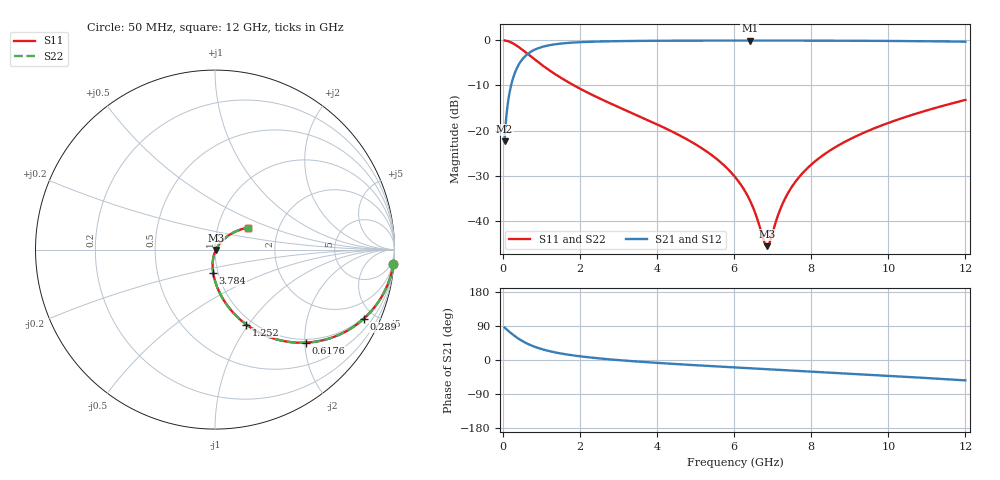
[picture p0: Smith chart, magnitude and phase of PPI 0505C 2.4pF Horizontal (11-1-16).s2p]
# MHz S MA R 50
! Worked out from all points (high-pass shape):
!   1601 points, 50 MHz to 12 GHz, reference 50 ohm
!   highest |S21| = -0.05 dB at 6.406 GHz (marker M1); lowest = -22.4 dB at 50 MHz (marker M2)
!   |S21| within 3 dB of the highest: 644.9 MHz to end of sweep
!   lowest |S11| = -45.6 dB at 6.854 GHz (marker M3), VSWR 1.01, Z = 50.5 - j0.228 ohm
!   |S11| at or under -10 dB: 1.851 GHz to end of sweep
!   |S22| runs from -45.6 to 0.0 dB; largest |S21 - S12| = 0
!   S11 on the Smith chart (normalised r, x): 50 MHz: 1, -25; 289 MHz: 0.93, -4.34; 617.6 MHz: 0.93, -2.02; 1.252 GHz: 0.93, -0.98; 3.784 GHz: 0.95, -0.25; 12 GHz: 1.39, +0.36
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50  0.9971 -4.6  0.07629 85.4  0.07629 85.4  0.9971 -4.6
169.5  0.9679 -15.2  0.2512 74.8  0.2512 74.8  0.9679 -15.2
289  0.9142 -24.9  0.4048 65.0  0.4048 65.0  0.9142 -24.9
438.375  0.8293 -35.5  0.5579 54.5  0.5579 54.5  0.8293 -35.5
617.625  0.7242 -45.7  0.6884 44.2  0.6884 44.2  0.7242 -45.7
908.9062  0.5781 -57.8  0.8143 32.1  0.8143 32.1  0.5781 -57.8
1252.469  0.4529 -67.3  0.8894 22.4  0.8894 22.4  0.4529 -67.3
2044.156  0.2856 -80.2  0.9556 9.3  0.9556 9.3  0.2856 -80.2
3784.375  0.1293 -94.5  0.9877 -6.1  0.9877 -6.1  0.1293 -94.5
4038.312  0.1153 -95.9  0.9893 -7.8  0.9893 -7.8  0.1153 -95.9
5255.719  0.05998 -101.1  0.9935 -15.3  0.9935 -15.3  0.05998 -101.1
6025  0.03063 -100.6  0.9944 -19.6  0.9944 -19.6  0.03063 -100.6
6405.906  0.01704 -94.7  0.9945 -21.7  0.9945 -21.7  0.01704 -94.7
6779.344  0.005898 -52.2  0.9944 -23.8  0.9944 -23.8  0.005898 -52.2
6854.031  0.00523 -25.5  0.9943 -24.2  0.9943 -24.2  0.00523 -25.5
6928.719  0.00586 1.3  0.9943 -24.6  0.9943 -24.6  0.00586 1.3
7167.719  0.01239 38.2  0.9941 -25.9  0.9941 -25.9  0.01239 38.2
7384.312  0.01975 46.6  0.9938 -27.1  0.9938 -27.1  0.01975 46.6
8019.156  0.04255 51.4  0.9927 -30.6  0.9927 -30.6  0.04255 51.4
8848.188  0.07395 49.8  0.9903 -35.2  0.9903 -35.2  0.07395 49.8
10013.31  0.122 44.8  0.9847 -41.8  0.9847 -41.8  0.122 44.8
12000  0.2186 33.9  0.9662 -53.8  0.9662 -53.8  0.2186 33.9
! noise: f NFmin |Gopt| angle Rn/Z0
50  0.000729  0.9401  1.976  0.002718
1372  0.005679  0.7605  5.93  0.004794
2701  0.009231  0.7173  10.36  0.006405
4031  0.01243  0.6927  14.85  0.007754
5360  0.01549  0.6776  19.3  0.009029
6682  0.01853  0.6688  23.65  0.01032
8012  0.02165  0.6649  27.94  0.01169
9341  0.02493  0.6652  32.13  0.01322
1.067e+04  0.02843  0.6689  36.2  0.01497
1.2e+04  0.03224  0.6759  40.17  0.01701
